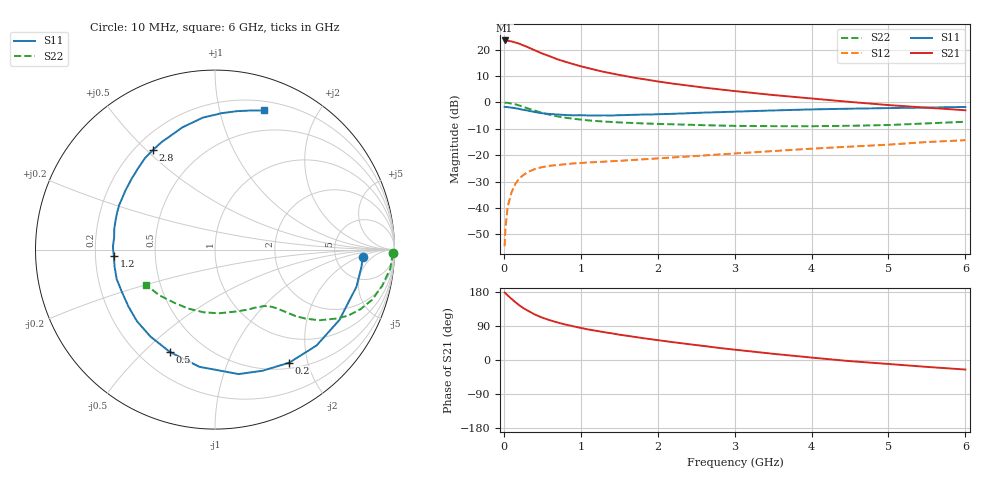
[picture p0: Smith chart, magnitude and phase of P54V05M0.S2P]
! SIEMENS Small Signal Semiconductors
! BFP183
! Si NPN RF Bipolar Junction Transistor in SOT143
! VCE = 4 V  IC = 5 mA
! Common Emitter S-Parameters:  March  1996
# GHz  S  MA  R  50
!  f  S11  S21  S12  S22
! GHz  MAG  ANG  MAG  ANG  MAG  ANG  MAG  ANG
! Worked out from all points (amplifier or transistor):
!   36 points, 10 MHz to 6 GHz, reference 50 ohm
!   highest |S21| = 23.5 dB at 10 MHz (marker M1)
!   |S21| within 3 dB of that: start of sweep to 346.9 MHz
!   unconditionally stable (mu >= 1): 1.577 GHz to 5.635 GHz
!   at 250 MHz: K = 0.20, MSG = 24.6 dB, |S12| = -27.6 dB
!   at 1.4 GHz: K = 0.94, MSG = 16.6 dB, |S12| = -22.3 dB
!   at 6 GHz: K = 0.94, MSG = 5.7 dB, |S12| = -14.3 dB
!   lowest NFmin = 1.15 dB at 450 MHz
!   S11 on the Smith chart (normalised r, x): 10 MHz: 9.65, -2.59; 200 MHz: 0.58, -1.70; 500 MHz: 0.32, -0.60; 1.2 GHz: 0.28, -0.03; 2.8 GHz: 0.27, +0.53; 6 GHz: 0.29, +1.37
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0.01  0.8238 -3.0  14.9 178.2  0.0019 85.1  0.9932 -1.2
0.02  0.8219 -6.4  14.88 176.6  0.004 83.7  0.9882 -2.5
0.05  0.8149 -14.7  14.78 170.5  0.0106 84.2  0.9822 -6.2
0.1  0.7962 -29.5  14.28 161.3  0.0199 75.0  0.9532 -12.2
0.15  0.7783 -43.3  13.63 152.6  0.0288 67.8  0.9192 -17.7
0.2  0.7537 -56.7  12.94 144.6  0.0362 61.9  0.8758 -22.3
0.25  0.725 -68.6  12.08 137.4  0.0418 56.9  0.828 -26.4
0.3  0.7058 -79.3  11.31 131.5  0.0471 52.6  0.7797 -29.5
0.4  0.6588 -97.6  9.746 120.4  0.0547 45.8  0.7008 -34.2
0.5  0.6236 -113.7  8.422 111.7  0.0598 40.3  0.6345 -37.3
0.6  0.6033 -126.6  7.448 104.8  0.0631 37.2  0.5822 -39.5
0.7  0.5903 -137.4  6.533 98.9  0.0654 34.8  0.5428 -40.8
0.9  0.5701 -154.9  5.323 89.1  0.0699 31.6  0.4913 -42.8
1.1  0.5676 -170.1  4.455 80.5  0.0732 30.5  0.457 -44.6
1.2  0.5651 -176.2  4.097 77.1  0.0741 29.7  0.4451 -45.6
1.7  0.5834 159.2  2.934 61.0  0.0818 30.5  0.4072 -51.5
2.2  0.609 140.0  2.267 47.0  0.0911 31.1  0.3854 -59.0
2.8  0.6544 121.7  1.769 31.8  0.1035 31.4  0.3654 -70.5
3.5  0.7048 104.9  1.382 16.4  0.12 30.5  0.3556 -86.5
4.5  0.761 87.2  1.023 -3.0  0.1456 26.7  0.3609 -114.5
5.5  0.8 75.6  0.795 -18.2  0.1779 22.0  0.401 -140.5
6  0.8218 70.6  0.711 -25.2  0.1926 18.0  0.4307 -152.6
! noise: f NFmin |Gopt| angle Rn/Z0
0.45  1.15  0.25  40  0.26
0.9  1.2  0.25  93  0.22
1.8  1.95  0.32  170  0.13
